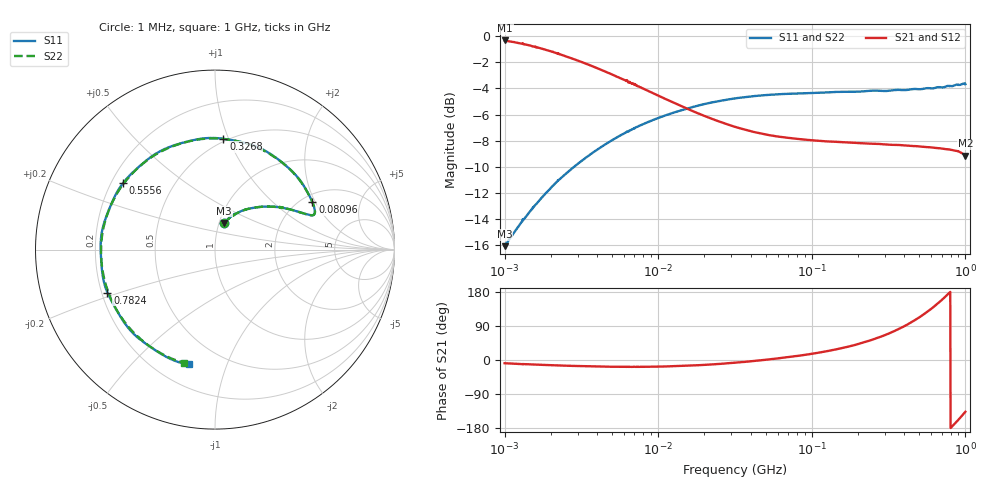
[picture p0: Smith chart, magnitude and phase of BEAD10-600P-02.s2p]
!s-Parameter Generated by FASTRON Sdn. Bhd.
!FASTRON P/N : BEAD/10-600P
!Vector Network Analyser E5071C,MY46733604,B.14.02
!Date: Mon Jul 31 13:17:02 2023
!Data & Calibration Information:
!Freq	S11:SOLT2(ON)	S21:SOLT2(ON)	S12:SOLT2(ON)	S22:SOLT2(ON)
!PortZ  Port1:50+j0  Port2:50+j0
!When reading, reference impedance value at option line is always used.
! Remarks : This data is being provided solely for informational purposes.
# Hz S dB R 50
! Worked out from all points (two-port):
!   1601 points, 1 MHz to 1 GHz, reference 50 ohm
!   highest |S21| = -0.32 dB at 1.01 MHz (marker M1); lowest = -9.2 dB at 1 GHz (marker M2)
!   |S21| within 3 dB of the highest: start of sweep to 5.954 MHz
!   lowest |S11| = -16.1 dB at 1 MHz (marker M3), VSWR 1.37, Z = 52.8 + j16.1 ohm
!   |S11| at or under -10 dB: start of sweep to 2.84 MHz
!   |S22| runs from -16.1 to -3.7 dB; largest |S21 - S12| = 0.0091
!   S11 on the Smith chart (normalised r, x): 1 MHz: 1.06, +0.32; 80.96 MHz: 2.28, +1.89; 326.8 MHz: 0.48, +0.96; 555.6 MHz: 0.25, +0.31; 782.4 MHz: 0.22, -0.18; 1 GHz: 0.33, -0.74
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1000000  -16.09 71.1  -0.33 -8.6  -0.34 -8.6  -16.13 71.0
1010197  -15.99 71.0  -0.32 -8.7  -0.33 -8.7  -16.05 71.0
1919221  -11.84 56.3  -1.09 -13.4  -1.09 -13.4  -11.86 56.1
3167252  -9.55 45.2  -1.98 -16.2  -1.97 -16.2  -9.56 45.2
1.002882e7  -6.26 26.9  -4.55 -17.5  -4.55 -17.4  -6.26 26.8
3.163788e7  -4.76 19.4  -6.94 -7.2  -6.94 -7.1  -4.77 19.3
8.095745e7  -4.39 25.9  -7.87 10.9  -7.86 10.9  -4.38 25.7
1.00144e8  -4.36 29.9  -7.97 16.4  -7.97 16.4  -4.35 29.8
1.446202e8  -4.27 40.4  -8.09 28.2  -8.08 28.2  -4.29 40.1
1.997956e8  -4.25 53.7  -8.18 41.8  -8.18 41.9  -4.25 53.5
2.531682e8  -4.17 67.4  -8.24 54.8  -8.24 54.8  -4.22 66.7
3.171813e8  -4.18 83.2  -8.31 69.9  -8.30 69.9  -4.18 82.7
3.267869e8  -4.16 85.7  -8.32 72.1  -8.31 72.2  -4.18 85.2
3.81318e8  -4.12 99.6  -8.35 84.8  -8.34 84.9  -4.15 98.9
4.386022e8  -4.08 114.0  -8.41 98.2  -8.40 98.3  -4.12 113.4
4.939769e8  -4.06 128.2  -8.44 110.9  -8.43 111.0  -4.08 127.4
5.555784e8  -3.98 144.0  -8.50 125.2  -8.49 125.3  -4.05 143.1
6.698054e8  -3.90 173.2  -8.58 151.2  -8.57 151.3  -3.96 172.0
7.824034e8  -3.80 -158.2  -8.67 176.5  -8.67 176.6  -3.88 -159.5
8.746054e8  -3.71 -134.7  -8.79 -163.1  -8.78 -163.0  -3.78 -136.4
9.446788e8  -3.69 -117.3  -8.94 -148.1  -8.94 -148.1  -3.72 -118.8
1e9  -3.68 -102.8  -9.15 -136.6  -9.14 -136.4  -3.69 -105.1
